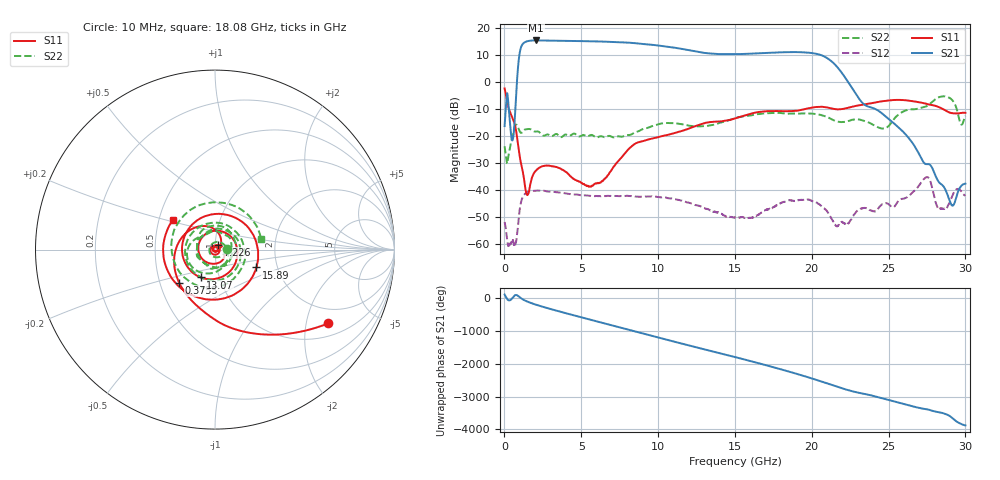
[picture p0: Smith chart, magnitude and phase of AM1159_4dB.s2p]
!Keysight Technologies,N5245B,MY58422270,A.16.20.02
!Date: Tuesday, December 10, 2024 23:19:40
!Correction: S11(C  2-Port  )
!S21(C  2-Port  )
!S12(C  2-Port  )
!S22(C  2-Port  )
!S2P File: Measurements: S11, S21, S12, S22:
# Hz S  dB  R 50
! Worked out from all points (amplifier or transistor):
!   6401 points, 10 MHz to 30 GHz, reference 50 ohm
!   highest |S21| = 15.2 dB at 2.053 GHz (marker M1)
!   |S21| within 3 dB of that: 1.052 GHz to 11.43 GHz (10.38 GHz wide, 166 % of centre)
!   unconditionally stable (mu >= 1): start of sweep to end of sweep
!   at 5.005 GHz: K = 10.92, MAG = 15.0 dB, |S12| = -41.9 dB
!   at 15.01 GHz: K = 44.77, MAG = 10.6 dB, |S12| = -50.0 dB
!   at 30 GHz: K = 4197.36, MAG = -37.0 dB, |S12| = -42.0 dB
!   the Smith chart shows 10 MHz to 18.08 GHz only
!   S11 on the Smith chart (normalised r, x): 10 MHz: 1.42, -2.68; 375.5 MHz: 0.63, -0.25; 7.226 GHz: 1.03, +0.05; 13.07 GHz: 0.81, -0.26; 15.89 GHz: 1.56, -0.33; 18.08 GHz: 0.59, +0.21
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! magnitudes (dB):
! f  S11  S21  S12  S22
! 10 MHz  -2.5  -16.4  -51.7  -23.8
! 202.1 MHz  -8.2  -4.9  -59.2  -29.8
! 375.5 MHz  -11.3  -16.2  -59.9  -23.8
! 562.9 MHz  -13.8  -20.8  -58.7  -18.8
! 989.4 MHz  -27.3  10.6  -47.2  -18.3
! 1.444 GHz  -41.5  14.9  -40.8  -17.5
! 2.053 GHz  -32.8  15.2  -40.2  -18.4
! 5.01 GHz  -37.3  15.0  -41.9  -19.8
! 7.226 GHz  -30.4  14.7  -42.1  -20.4
! 10.01 GHz  -20.4  13.4  -42.5  -15.7
! 13.07 GHz  -15.2  10.6  -46.8  -16.4
! 15.01 GHz  -13.6  10.2  -50.0  -13.5
! 15.89 GHz  -12.0  10.3  -50.2  -12.5
! 18.08 GHz  -10.9  10.9  -44.5  -11.6
! 20 GHz  -9.5  10.6  -44.0  -11.8
! 21.63 GHz  -10.2  5.6  -53.3  -14.7
! 25 GHz  -6.9  -13.7  -45.2  -16.3
! 27.47 GHz  -8.1  -30.4  -35.2  -9.0
! 28.27 GHz  -9.3  -37.0  -47.0  -5.7
! 29.11 GHz  -11.6  -45.5  -42.5  -6.6
! 29.7 GHz  -11.5  -38.6  -40.2  -15.6
! 30 GHz  -11.5  -37.6  -42.0  -12.6
